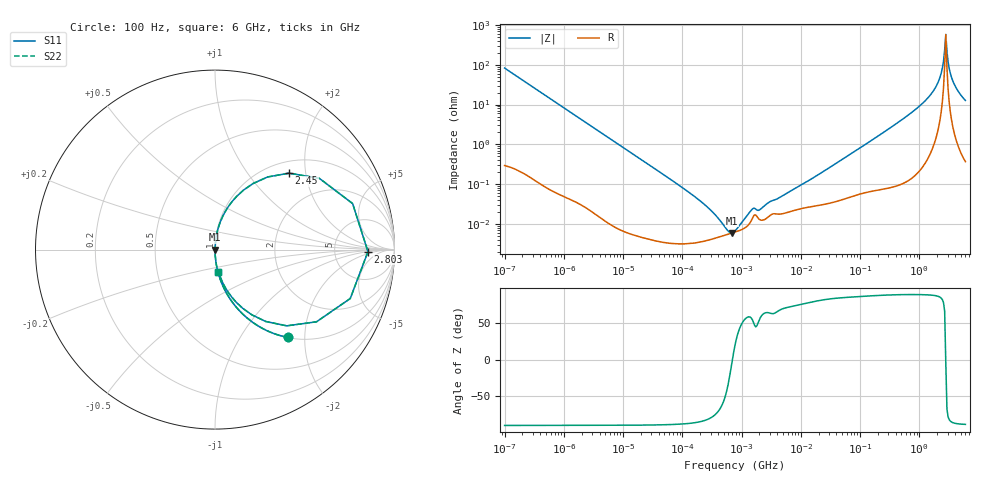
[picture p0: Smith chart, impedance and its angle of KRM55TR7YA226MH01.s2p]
!Murata Part Number: KRM55TR7YA226MH01
!These Parameters are Measured in Series Mode Connection
!Data Generated on Jan 08, 2026
!  o--ll--o
!Port1  Port2
!  o------o
!Operation Temp=25[degC], DC Bias Voltage=0[V]
!Freq. Start=100[Hz] Stop=6[GHz] 401[Steps]
# Hz S RI R 50
!Freq.(Hz) S11(Real) S11(Imag) S21(Real) S21(Imag) S12(Real) S12(Imag) S22(Real) S22(Imag)
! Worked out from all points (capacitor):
!   401 points, 100 Hz to 6 GHz, reference 50 ohm
!   read as one part in series: C = 19.3 uF near 109 Hz
!   lowest |Z| = 5.94 mohm at 677.2 kHz (marker M1)
!   series resonance near 700.4 kHz, so ESL is about 2.7 nH
!   S11 on the Smith chart (normalised r, x): 100 Hz: 1.01, -1.65; 2.45 GHz: 1.23, +1.62; 2.803 GHz: 12, -1; 6 GHz: 1.01, -0.25
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100  0.4055 -0.4892  0.5945 0.4892  0.5945 0.4892  0.4055 -0.4892
306  0.0692 -0.2515  0.9308 0.2515  0.9308 0.2515  0.0692 -0.2515
2008  0.00201 -0.0414  0.998 0.0414  0.998 0.0414  0.00201 -0.0414
40335  4.05e-05 -0.00208  1 0.00208  1 0.00208  4.05e-05 -0.00208
202169  3.55e-05 -0.000374  1 0.000374  1 0.000374  3.55e-05 -0.000374
473344  5e-05 -9.06e-05  1 9.06e-05  1 9.06e-05  5e-05 -9.06e-05
677235  5.89e-05 -7.4e-06  0.9999 7.4e-06  0.9999 7.4e-06  5.89e-05 -7.4e-06
774597  6.27e-05 2.24e-05  0.9999 -2.24e-05  0.9999 -2.24e-05  6.27e-05 2.24e-05
968953  7.07e-05 7.37e-05  0.9999 -7.37e-05  0.9999 -7.37e-05  7.07e-05 7.37e-05
1516199  0.000137 0.000193  0.9999 -0.000193  0.9999 -0.000193  0.000137 0.000193
2074311  0.000127 0.000197  0.9999 -0.000197  0.9999 -0.000197  0.000127 0.000197
1.555665e7  0.000277 0.00137  0.9997 -0.00137  0.9997 -0.00137  0.000277 0.00137
3.124326e8  0.00144 0.0251  0.9986 -0.0251  0.9986 -0.0251  0.00144 0.0251
9.569533e8  0.00921 0.0847  0.9908 -0.0847  0.9908 -0.0847  0.00921 0.0847
1.712697e9  0.0519 0.2026  0.9481 -0.2026  0.9481 -0.2026  0.0519 0.2026
2.142435e9  0.1589 0.3314  0.8411 -0.3314  0.8411 -0.3314  0.1589 0.3314
2.450438e9  0.413 0.4259  0.587 -0.4259  0.587 -0.4259  0.413 0.4259
2.802721e9  0.8523 -0.0114  0.1477 0.0114  0.1477 0.0114  0.8523 -0.0114
3.065283e9  0.5657 -0.4022  0.4343 0.4022  0.4343 0.4022  0.5657 -0.4022
3.352442e9  0.2833 -0.4007  0.7167 0.4007  0.7167 0.4007  0.2833 -0.4007
4.009986e9  0.0922 -0.2633  0.9078 0.2633  0.9078 0.2633  0.0922 -0.2633
6e9  0.0193 -0.1236  0.9807 0.1236  0.9807 0.1236  0.0193 -0.1236
